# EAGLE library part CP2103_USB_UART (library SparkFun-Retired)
Single-Chip USB to UART Bridge Source: www.silabs.com .. CP2103.pdf. Spark Fun Electronics SKU : COM-00309 Retired: IC-00866
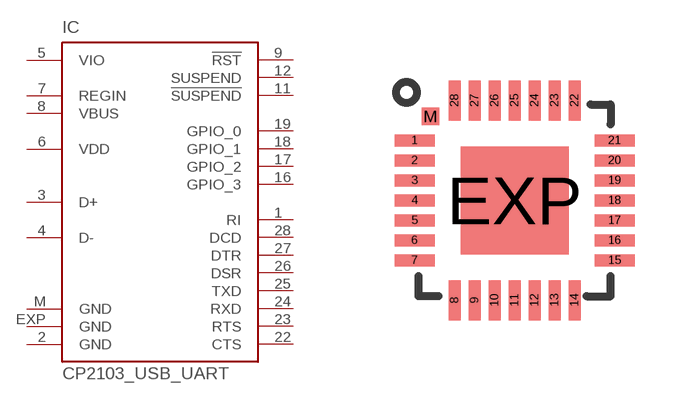
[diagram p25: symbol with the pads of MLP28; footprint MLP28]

Designator prefix IC

## CP2103_USB_UART (PROD_ID: COM-00309; VALUE: CP2103)  [MLP28]
1  RI  in
2  GND  pwr
3  D+
4  D-
5  VIO  pwr
6  VDD  pwr
7  REGIN  pas
8  VBUS  in
9  !RST
11  !SUSPEND  out
12  SUSPEND  out
16  GPIO_3
17  GPIO_2
18  GPIO_1
19  GPIO_0
22  CTS  in
23  RTS  out
24  RXD  in
25  TXD  out
26  DSR  in
27  DTR  out
28  DCD  in
EXP  GND  pwr
M  GND  pwr

## Footprint MLP28 (pad centres in mm)
MLP 28 Source: www.silabs.com .. CP2101.pdf
smd 1 x 0.3: 1 -2.5,1.5; 2 -2.5,1; 3 -2.5,0.5; 4 -2.5,0; 5 -2.5,-0.5; 6 -2.5,-1; 7 -2.5,-1.5; 15 2.5,-1.5; 16 2.5,-1; 17 2.5,-0.5; 18 2.5,0; 19 2.5,0.5; 20 2.5,1; 21 2.5,1.5
smd 0.3 x 1: 8 -1.5,-2.5; 9 -1,-2.5; 10 -0.5,-2.5; 11 0,-2.5; 12 0.5,-2.5; 13 1,-2.5; 14 1.5,-2.5; 22 1.5,2.5; 23 1,2.5; 24 0.5,2.5; 25 0,2.5; 26 -0.5,2.5; 27 -1,2.5; 28 -1.5,2.5
smd 2.7 x 2.7: EXP 0,0
smd 0.435 x 0.435: M -2.103,2.103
